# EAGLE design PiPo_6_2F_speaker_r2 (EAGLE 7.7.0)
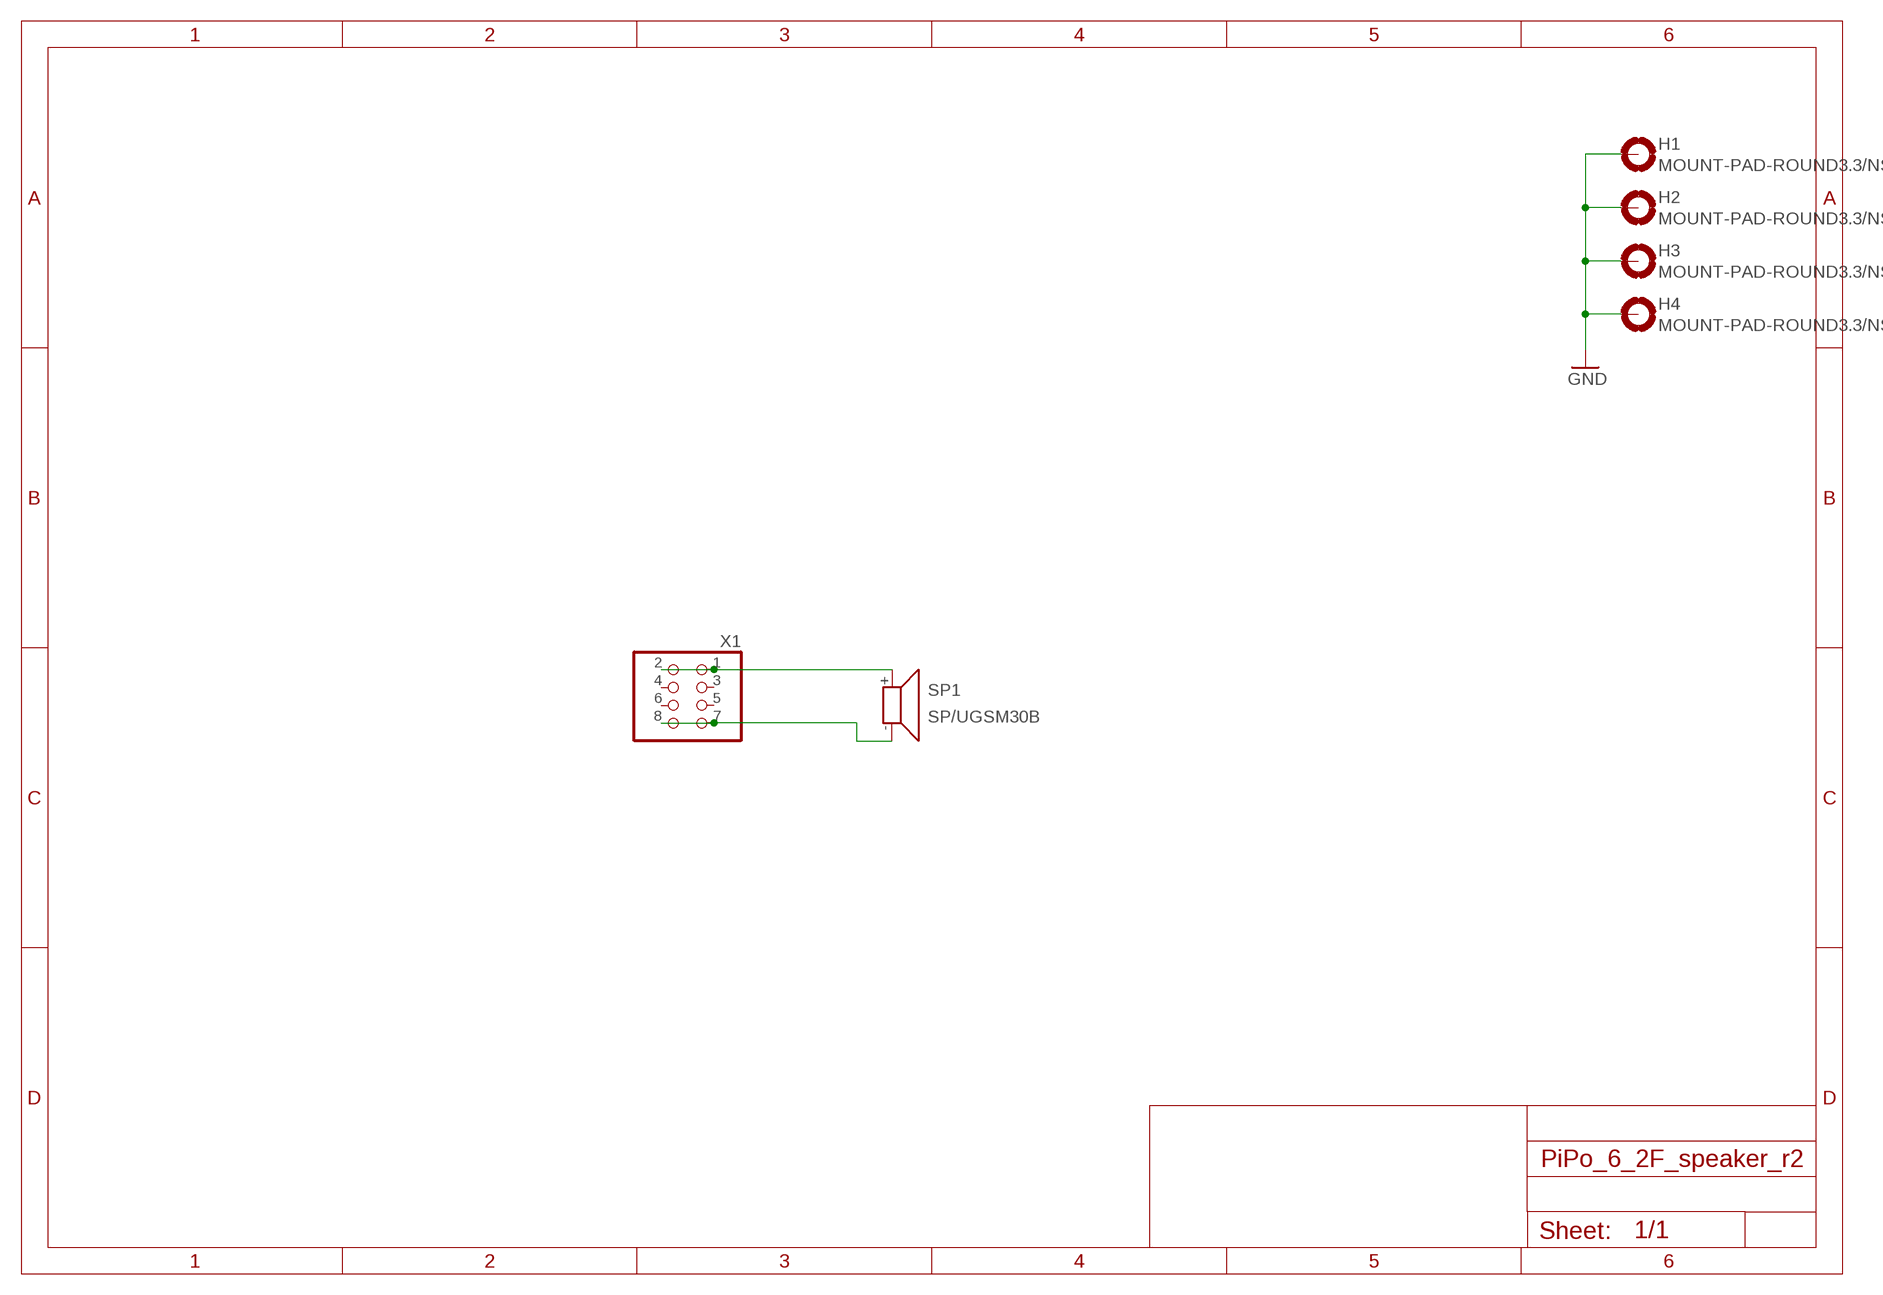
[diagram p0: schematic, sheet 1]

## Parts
H1  MOUNT-PAD-ROUND3.3/NS  [3,3-PAD/NS]
H2  MOUNT-PAD-ROUND3.3/NS  [3,3-PAD/NS]
H3  MOUNT-PAD-ROUND3.3/NS  [3,3-PAD/NS]
H4  MOUNT-PAD-ROUND3.3/NS  [3,3-PAD/NS]
SP1  SP/UGSM30B  [UGSM30B]
X1  PINHD-2X4SKT/SMT/WB  [2X04SKT/SMT/WB]

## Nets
GND: H1.B3,3(MOUNT) H2.B3,3(MOUNT) H3.B3,3(MOUNT) H4.B3,3(MOUNT)
N$1: SP1.+ X1.1 X1.2
N$2: SP1.- X1.7 X1.8
Unconnected: X1.3 X1.4 X1.5 X1.6

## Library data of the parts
H1-H4 = my-holes:MOUNT-PAD-ROUND: MOUNTING PAD, round
SP1 = my-speaker:SP/: Speaker 13 x 13mm, 8 Ohm, 0.7W
X1 = pinhead:PINHD-2X4: PIN HEADER

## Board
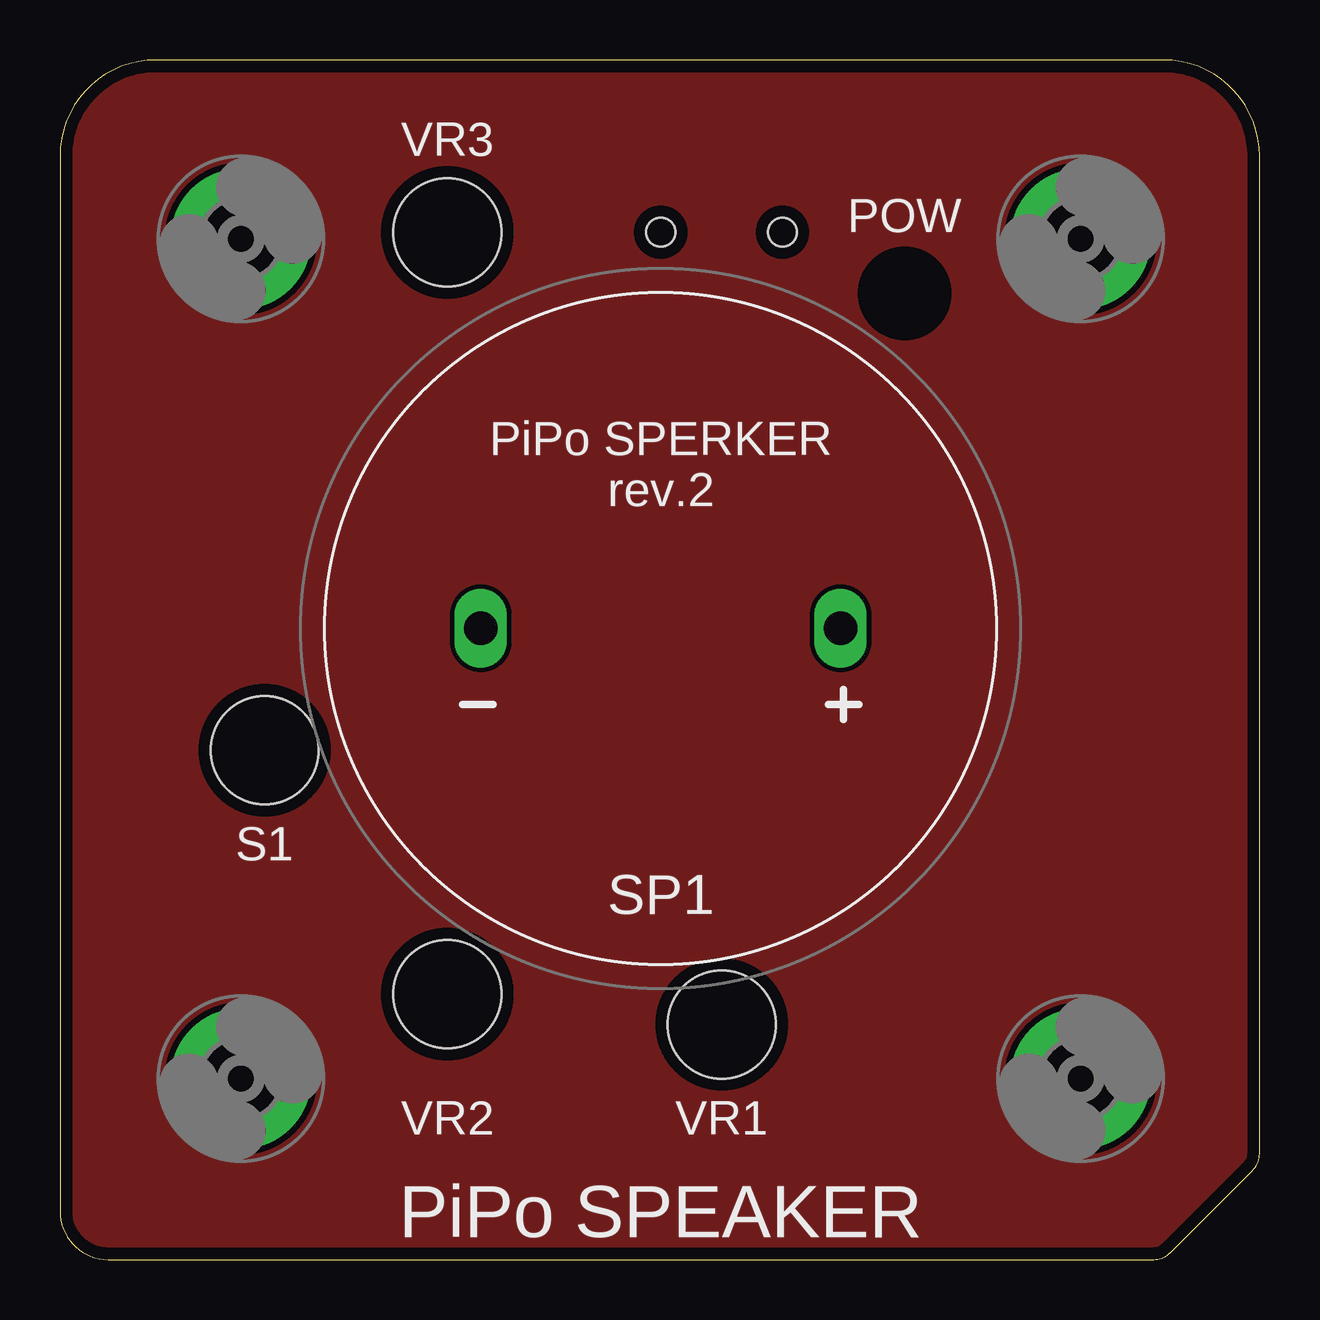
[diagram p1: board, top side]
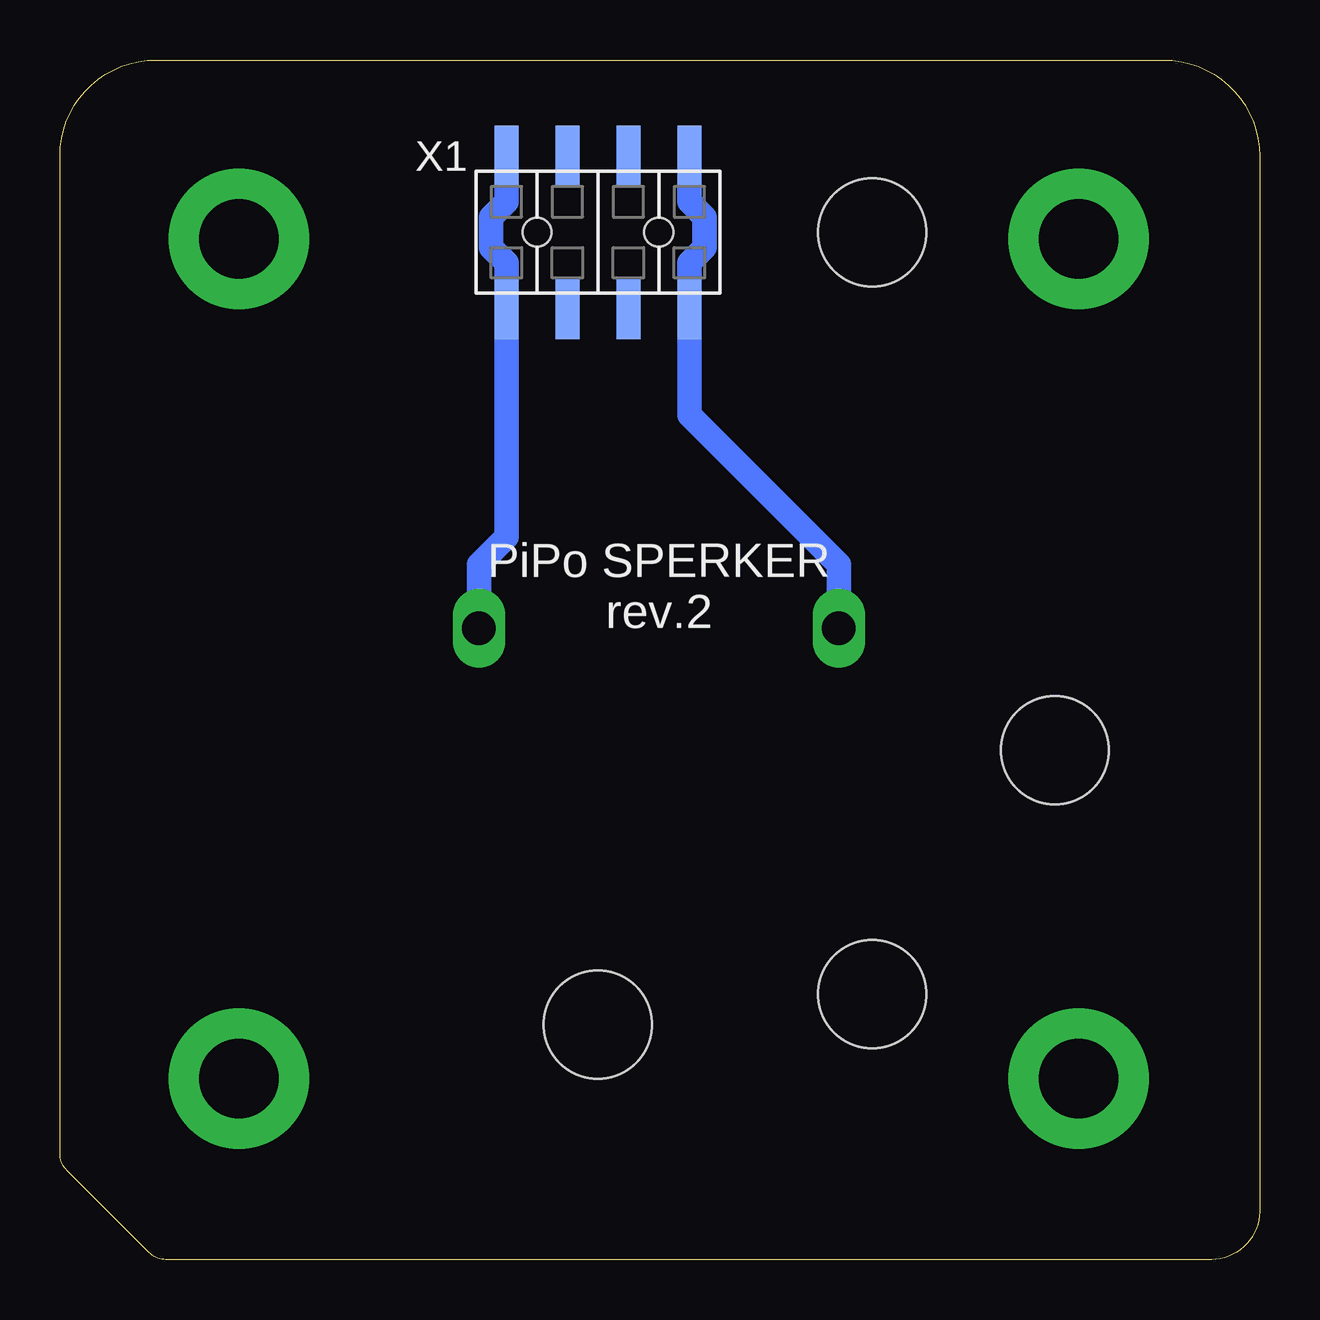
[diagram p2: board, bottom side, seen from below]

Size 50 x 50 mm. Coordinates in mm from the lower left corner, seen from the top.
Outline: 0,46 0,2 arc90 2,0 45.59,0 arc45 46.29,0.29 49.71,3.71 arc45 50,4.41 50,46 arc90 46,50 4,50 arc90 0,46
Copper layers (1*16): Top 0.035mm / dielectric 1.5mm / Bottom 0.035mm
Design rules "default *": minimum track width 10mil, minimum drill 24mil, track to track 8mil, track to pad 8mil, pad to pad 8mil, via to via 8mil, smd to smd 8mil, copper to edge 20mil, drill to drill 8mil, minimum pad ring 10mil, minimum via ring 8mil, stop-mask expansion 4mil, vias tented up to drill 0mil, thermal gap 10mil
Holes 4.5 mm at 27.58,9.8 16.15,11.07 8.53,21.23 16.15,42.82
tRestrict: area 33.4,38.5 to 37,42.1

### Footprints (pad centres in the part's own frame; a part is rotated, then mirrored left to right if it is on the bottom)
3,3-PAD/NS = drill 3.3 pad 5.842: B3,3 0,0
UGSM30B = drill 1.4 pad 2.184 long: + -7.5,0; - 7.5,0
2X04SKT/SMT/WB = smd 1 x 2.5: 1 -3.81,-3.195; 2 -3.81,3.195; 3 -1.27,-3.195; 4 -1.27,3.195; 5 1.27,-3.195; 6 1.27,3.195; 7 3.81,-3.195; 8 3.81,3.195 | hole 1.2: -2.54,0; 2.54,0

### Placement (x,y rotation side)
H1  42.54,7.54 0 top
H2  42.54,42.54 0 top
H3  7.54,42.54 0 top
H4  7.54,7.54 0 top
SP1  25.04,26.31 180 top
X1  27.58,42.82 0 bottom

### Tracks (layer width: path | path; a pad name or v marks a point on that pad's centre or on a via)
GND
  pour Top: 0,0 50,0 50,50 0,50
N$1
  Bottom 1.016: SP1.+ 32.54,28.97 31.39,30.12 X1.1 31.39,41.55 32.02,42.19 32.02,43.46 31.39,44.09 X1.2
N$2
  Bottom 1.016: SP1.- 17.54,28.97 23.77,35.2 X1.7 23.77,41.55 23.13,42.19 23.13,43.46 23.77,44.09 X1.8

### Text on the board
tPlace: VR3 | POW | PiPo SPERKER / rev.2 | S1 | VR2 | VR1 | PiPo SPEAKER
bPlace: PiPo SPERKER / rev.2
